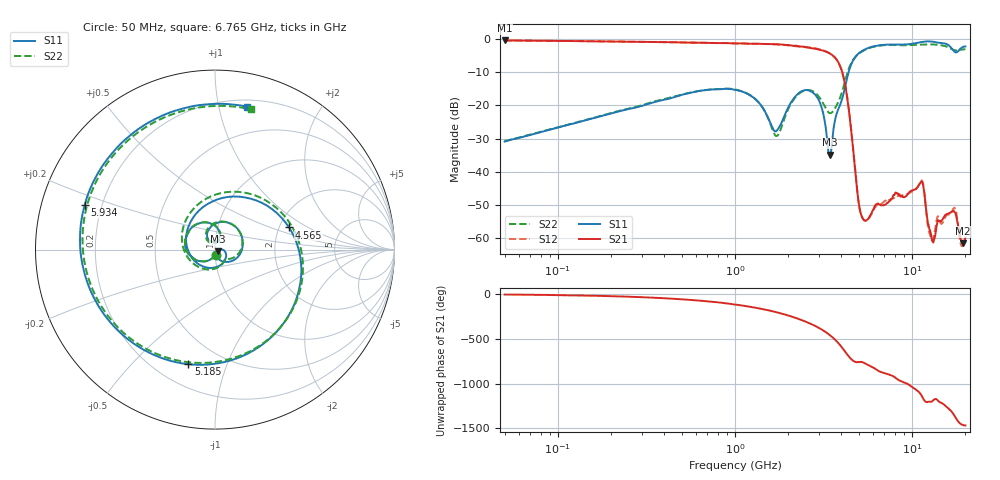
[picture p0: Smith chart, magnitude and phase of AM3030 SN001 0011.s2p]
# Hz S DB R 50
!freq MagS11 AngS11 MagS21 AngS21 MagS12 AngS12 MagS22 AngS22
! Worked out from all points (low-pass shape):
!   1601 points, 50 MHz to 20.05 GHz, reference 50 ohm
!   highest |S21| = -0.38 dB at 50 MHz (marker M1); lowest = -61.5 dB at 19.39 GHz (marker M2)
!   |S21| within 3 dB of the highest: start of sweep to 3.131 GHz
!   lowest |S11| = -34.8 dB at 3.434 GHz (marker M3), VSWR 1.04, Z = 51.5 - j1.06 ohm
!   |S11| at or under -10 dB: start of sweep to 4.385 GHz
!   |S22| runs from -30.6 to -1.5 dB; largest |S21 - S12| = 0.017
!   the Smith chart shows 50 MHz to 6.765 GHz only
!   S11 on the Smith chart (normalised r, x): 50 MHz: 1.00, -0.06; 4.565 GHz: 2.26, +0.69; 5.185 GHz: 0.33, -0.74; 5.934 GHz: 0.14, +0.16; 6.765 GHz: 0.25, +1.22
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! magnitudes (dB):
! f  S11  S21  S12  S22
! 50 MHz  -30.9  -0.4  -0.4  -30.6
! 135.9 MHz  -24.8  -0.6  -0.6  -24.7
! 369.6 MHz  -18.7  -0.9  -0.9  -18.5
! 1.005 GHz  -15.3  -1.3  -1.3  -15.2
! 1.356 GHz  -19.0  -1.4  -1.4  -18.9
! 1.717 GHz  -27.7  -1.5  -1.6  -29.2
! 2.182 GHz  -17.4  -2.0  -2.1  -17.7
! 2.722 GHz  -15.9  -2.8  -2.6  -15.6
! 3.081 GHz  -20.4  -3.3  -3.2  -18.5
! 3.434 GHz  -34.8  -4.3  -4.3  -22.3
! 4.065 GHz  -17.4  -10.4  -10.5  -15.2
! 4.565 GHz  -7.3  -28.8  -28.6  -7.0
! 4.939 GHz  -4.6  -47.0  -47.1  -4.7
! 5.185 GHz  -3.7  -53.2  -53.2  -3.8
! 5.934 GHz  -2.3  -52.3  -52.6  -2.4
! 6.765 GHz  -1.8  -50.1  -49.6  -1.9
! 7.402 GHz  -1.6  -48.9  -48.6  -1.7
! 11.3 GHz  -0.9  -42.9  -42.7  -1.6
! 12.84 GHz  -0.7  -59.0  -59.9  -1.5
! 17.32 GHz  -3.7  -51.9  -50.9  -3.3
! 19.39 GHz  -2.4  -61.5  -62.0  -3.1
! 20.05 GHz  -2.2  -59.8  -60.0  -3.0
